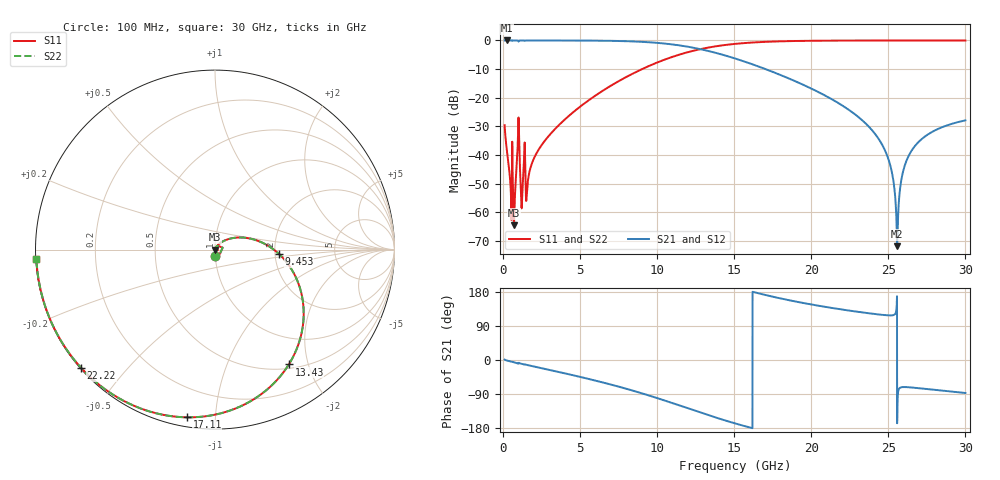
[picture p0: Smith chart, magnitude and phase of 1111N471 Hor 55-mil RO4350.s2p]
# GHz S MA R 50
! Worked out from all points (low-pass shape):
!   3201 points, 100 MHz to 30 GHz, reference 50 ohm
!   highest |S21| = 0.00 dB at 268.2 MHz (marker M1); lowest = -71.9 dB at 25.57 GHz (marker M2)
!   |S21| within 3 dB of the highest: start of sweep to 12.77 GHz
!   lowest |S11| = -64.6 dB at 707.3 MHz (marker M3), VSWR 1.00, Z = 50.1 - j0.00659 ohm
!   |S11| at or under -10 dB: start of sweep to 9.024 GHz
!   |S22| runs from -64.6 to 0.0 dB; largest |S21 - S12| = 0
!   S11 on the Smith chart (normalised r, x): 100 MHz: 1.00, -0.07; 9.453 GHz: 2.10, -0.11; 13.43 GHz: 0.56, -1.69; 17.11 GHz: 0.05, -0.85; 22.22 GHz: 0.00, -0.38; 30 GHz: 0.00, -0.03
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0.1  0.03306 -88.5  0.9992 1.1  0.9992 1.1  0.03306 -88.5
0.2681875  0.01069 -89.8  0.9996 -1.6  0.9996 -1.6  0.01069 -89.8
0.5952188  0.01702 -16.1  0.9832 -4.8  0.9832 -4.8  0.01702 -16.1
0.7073438  0.0005903 -6.4  0.9993 -5.9  0.9993 -5.9  0.0005903 -6.4
0.9689688  0.02161 56.9  0.991 -9.2  0.991 -9.2  0.02161 56.9
1.202562  0.001166 -0.3  0.9987 -10.0  0.9987 -10.0  0.001166 -0.3
1.604344  0.003376 60.3  0.9989 -13.5  0.9989 -13.5  0.003376 60.3
2.501344  0.01484 65.2  0.9988 -21.6  0.9988 -21.6  0.01484 65.2
5.089563  0.07271 43.6  0.9956 -45.4  0.9956 -45.4  0.07271 43.6
9.453094  0.3567 -3.8  0.9308 -93.4  0.9308 -93.4  0.3567 -3.8
10.06978  0.4188 -11.7  0.9043 -101.4  0.9043 -101.4  0.4188 -11.7
13.43353  0.7606 -57.3  0.6434 -147.0  0.6434 -147.0  0.7606 -57.3
15.05  0.8708 -77.5  0.4845 -167.3  0.4845 -167.3  0.8708 -77.5
17.10562  0.9475 -99.5  0.3101 170.8  0.3101 170.8  0.9475 -99.5
20.03956  0.9871 -124.1  0.1426 146.3  0.1426 146.3  0.9871 -124.1
22.21666  0.9952 -138.6  0.06723 131.9  0.06723 131.9  0.9952 -138.6
24.02934  0.9972 -149.0  0.02535 121.8  0.02535 121.8  0.9972 -149.0
25.01978  0.9975 -154.2  0.008199 117.8  0.008199 117.8  0.9975 -154.2
25.57106  0.9975 -157.0  0.0002544 -166.9  0.0002544 -166.9  0.9975 -157.0
25.98219  0.9975 -159.0  0.005466 -71.4  0.005466 -71.4  0.9975 -159.0
26.63625  0.9974 -162.2  0.01331 -73.0  0.01331 -73.0  0.9974 -162.2
30  0.9965 -177.0  0.04016 -87.1  0.04016 -87.1  0.9965 -177.0
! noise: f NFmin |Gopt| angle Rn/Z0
0.1  0.0006655  0.7343  0.9275  0.0005002
3.417  0.008212  0.4138  27.43  0.002174
6.743  0.01475  0.3979  49.7  0.003375
10.06  0.02345  0.4595  67.79  0.005335
13.39  0.03817  0.5824  85.69  0.009489
16.7  0.06906  0.7365  105.8  0.01985
20.03  0.1529  0.8717  126.5  0.05293
23.35  0.5455  0.9617  145.6  0.2836
26.67  1.599  0.9861  162.3  0.6395
30  0.5789  0.9604  176.9  0.003735
